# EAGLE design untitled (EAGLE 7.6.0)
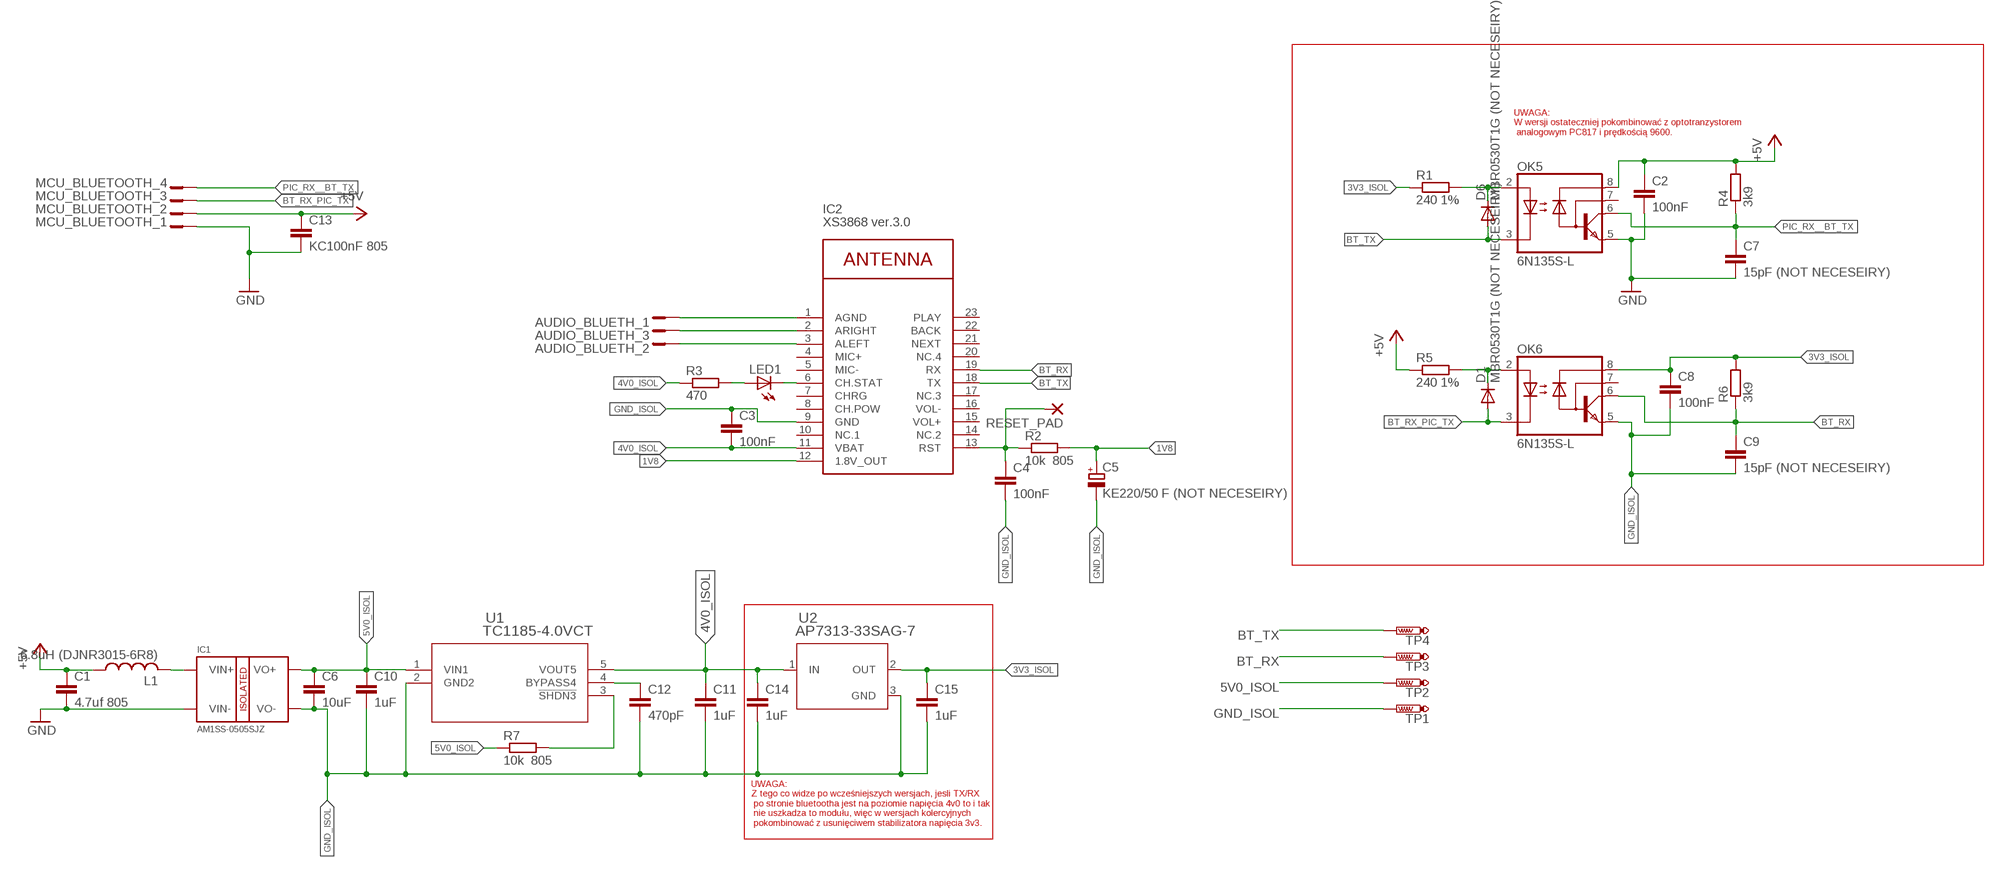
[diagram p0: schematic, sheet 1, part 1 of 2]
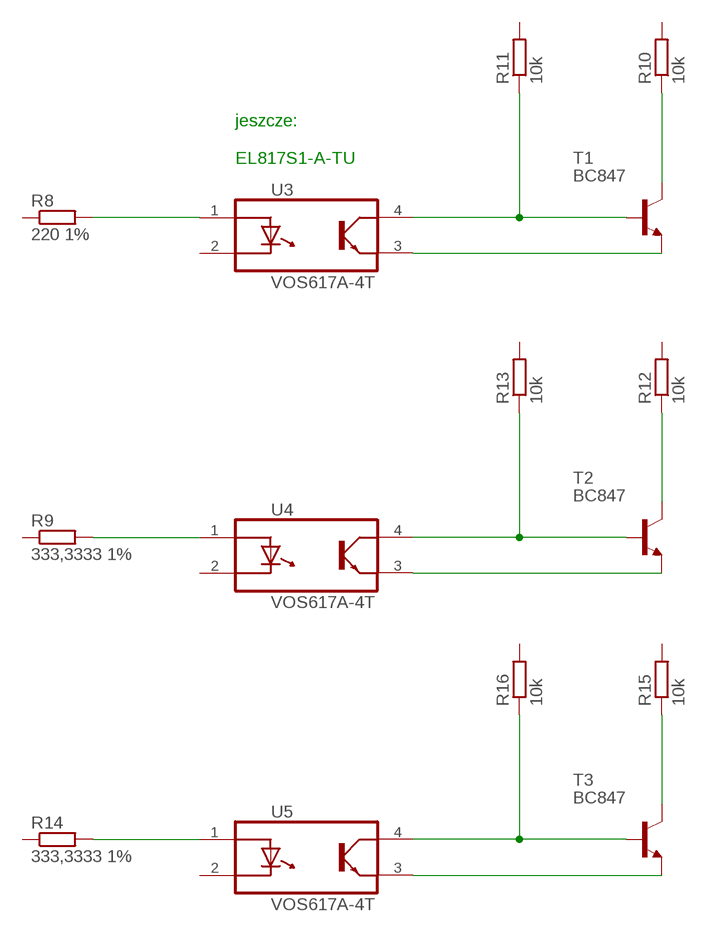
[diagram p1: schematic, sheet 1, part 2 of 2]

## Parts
AUDIO_BLUETH  JST_3_PIN_B3B-PH-KS  [B3B-PH-KS]
C1  4.7uf 805  C-EUC0805  [C0805]
C2  100nF  C-EUC0805  [C0805]
C3  100nF  C-EUC0805  [C0805]
C4  100nF  C-EUC0805  [C0805]
C5  KE220/50 F (NOT NECESEIRY)  CPOL-EUG  [PANASONIC_G]
C6  10uF  C-EUC0805  [C0805]
C7  15pF (NOT NECESEIRY)  C-EUC0805  [C0805]
C8  100nF  C-EUC0805  [C0805]
C9  15pF (NOT NECESEIRY)  C-EUC0805  [C0805]
C10  1uF  C-EUC0805  [C0805]
C11  1uF  C-EUC0805  [C0805]
C12  470pF  C-EUC0805  [C0805]
C13  KC100nF 805  C-EUC0805  [C0805]
C14  1uF  C-EUC0805  [C0805]
C15  1uF  C-EUC0805  [C0805]
D1  MBR0530T1G (NOT NECESEIRY)  MBR0520LT  [SOD123]
D6  MBR0530T1G (NOT NECESEIRY)  MBR0520LT  [SOD123]
IC1  AM1SS-0505SJZ  AM1SS-0503S-NZ  [SIP4]
IC2  XS3868 ver.3.0  WIRELESS-BLUETOOTH-XS3868  [WIRELESS-BLUETOOTH-XS3868]
L1  6.8uH (DJNR3015-6R8)  L-USL3230M  [L3230M]
LED1  LEDSMART-LED  [SMART-LED]
MCU_BLUETOOTH  JST_4_PIN_B4B-PH-KS  [B4B-PH-KS]
OK5  6N135S-L  6N135DIL8-SMD  [DIL8-SMD]
OK6  6N135S-L  6N135DIL8-SMD  [DIL8-SMD]
R1  240 1%  R-EU_M0805  [M0805]
R2  10k 805  R-EU_M0805  [M0805]
R3  470  R-EU_M0805  [M0805]
R4  3k9  R-EU_M0805  [M0805]
R5  240 1%  R-EU_M0805  [M0805]
R6  3k9  R-EU_M0805  [M0805]
R7  10k 805  R-EU_M0805  [M0805]
R8  220 1%  R-EU_M0805  [M0805]
R9  333,3333 1%  R-EU_M0805  [M0805]
R10  10k  R-EU_M0805  [M0805]
R11  10k  R-EU_M0805  [M0805]
R12  10k  R-EU_M0805  [M0805]
R13  10k  R-EU_M0805  [M0805]
R14  333,3333 1%  R-EU_M0805  [M0805]
R15  10k  R-EU_M0805  [M0805]
R16  10k  R-EU_M0805  [M0805]
RESET_PAD  SMD2  [SMD1,27-2,54]
T1  BC847  [SOT23]
T2  BC847  [SOT23]
T3  BC847  [SOT23]
TP1  PTR1B1,27  [B1,27]
TP2  PTR1B1,27  [B1,27]
TP3  PTR1B1,27  [B1,27]
TP4  PTR1B1,27  [B1,27]
U1  TC1185-4.0VCT  TC1185-X.XXCT713SOT-23-5_MC-M  [SOT-23-5_MC-M]
U2  AP7313-33SAG-7  [SOT-23]
U3  VOS617A-4T  [SOIC127P700X210-4N]
U4  VOS617A-4T  [SOIC127P700X210-4N]
U5  VOS617A-4T  [SOIC127P700X210-4N]

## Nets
1V8: C5.+ IC2.12(1.8V_OUT) R2.2
3V3_ISOL: C8.1 C15.1 OK6.8(VCC) R1.1 R6.2 U2.2(OUT)
4V0_ISOL: C3.2 C11.1 C14.1 IC2.11(VBAT) R3.1 U1.5(VOUT5) U2.1(IN)
5V0_ISOL: C6.1 C10.1 IC1.P$4(VO+) R7.1 TP2.TP U1.1(VIN1)
+5V: C1.1 C2.1 C13.1 L1.1 MCU_BLUETOOTH.P$2 OK5.8(VCC) R4.2 R5.1
AGND: AUDIO_BLUETH.P$1 IC2.1(AGND)
BT_LED: IC2.6(CH.STAT) LED1.B(C)
BT_RX: C9.1 IC2.19(RX) OK6.6(VO) R6.1 TP3.TP
BT_RX_PIC_TX: D1.A MCU_BLUETOOTH.P$3 OK6.3(C)
BT_TX: D6.A IC2.18(TX) OK5.3(C) TP4.TP
BTOUT_LEFT: AUDIO_BLUETH.P$2 IC2.3(ALEFT)
BTOUT_RIGHT: AUDIO_BLUETH.P$3 IC2.2(ARIGHT)
GND: C1.2 C2.2 C7.2 C13.2 IC1.P$1(VIN-) MCU_BLUETOOTH.P$1 OK5.5(GND)
GND_ISOL: C3.1 C4.2 C5.- C6.2 C8.2 C9.2 C10.2 C11.2 C12.2 C14.2 C15.2 IC1.P$3(VO-) IC2.9(GND) OK6.5(GND) TP1.TP U1.2(GND2) U2.3(GND)
N$1: IC1.P$2(VIN+) L1.2
N$2: D6.C OK5.2(A) R1.2
N$3: D1.C OK6.2(A) R5.2
N$4: C12.1 U1.4(BYPASS4)
N$5: LED1.A R3.2
N$6: R7.2 U1.3(!SHDN3)
N$7: R8.2 U3.1(A)
N$8: R9.2 U4.1(A)
N$9: R10.1 T1.3(C)
N$10: R11.1 T1.1(B) U3.4(CO)
N$11: T1.2(E) U3.3(E)
N$12: R12.1 T2.3(C)
N$13: R13.1 T2.1(B) U4.4(CO)
N$14: T2.2(E) U4.3(E)
N$15: R14.2 U5.1(A)
N$16: R15.1 T3.3(C)
N$17: R16.1 T3.1(B) U5.4(CO)
N$18: T3.2(E) U5.3(E)
PIC_RX__BT_TX: C7.1 MCU_BLUETOOTH.P$4 OK5.6(VO) R4.1
RST: C4.1 IC2.13(RST) R2.1 RESET_PAD.1(P)
Unconnected: IC2.4(MIC+) IC2.5(MIC-) IC2.7(CHRG) IC2.8(CH.POW) IC2.10(NC.1) IC2.14(NC.2) IC2.15(VOL+) IC2.16(VOL-) IC2.17(NC.3) IC2.20(NC.4) IC2.21(NEXT) IC2.22(BACK) IC2.23(PLAY) OK5.7(VB) OK6.7(VB) R8.1 R9.1 R10.2 R11.2 R12.2 R13.2 R14.1 R15.2 R16.2 U3.2(C) U4.2(C) U5.2(C)

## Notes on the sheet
- jeszcze:
  
  EL817S1-A-TU
- UWAGA:
  W wersji ostateczniej pokombinować z optotranzystorem
   analogowym PC817 i prędkością 9600.
- UWAGA:
  Z tego co widze po wcześniejszych wersjach, jesli TX/RX
   po stronie bluetootha jest na poziomie napięcia 4v0 to i tak
   nie uszkadza to modułu, więc w wersjach kolercyjnych
   pokombinować z usunięciwem stabilizatora napięcia 3v3.

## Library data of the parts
AUDIO_BLUETH = conn-JST:JST_3_PIN_
C1 C13 = rcl:C-EU: CAPACITOR, European symbol
C2-C4 C6-C12 C14 C15 = resistor:C-EU: CAPACITOR, European symbol
C5 = rcl:CPOL-EU: POLARIZED CAPACITOR, European symbol
D1 D6 = diode:MBR0520LT: SCHOTTKY BARRIER RECTIFIER
IC1 = DC-DC_converter:AM1SS
IC2 = diy-modules:WIRELESS-BLUETOOTH-XS3868: Bluetooth Stereo Audio Module based on OVC3860 chip More details available here: http://artofcircuits.com/product/bluetooth-2-0-edr-stereo-audio-ovc3860-module-model-xs-3868 Click here to find device on ebay.com
L1 = rcl:L-US: INDUCTOR, American symbol
LED1 = led:LED: LED
MCU_BLUETOOTH = conn-JST:JST_4_PIN_
OK5 OK6 = optocoupler:6N135: MOTOROLA OPTO COUPLER
R1-R16 = rcl:R-EU_: RESISTOR, European symbol
RESET_PAD = wirepad:SMD2: SMD PAD
T1-T3 = nxp_60:BC847: 45 V, 100 mA NPN general-purpose transistors NPN general-purpose transistor AAL Eindhoven MK
TP1-TP4 = testpad:PTR1: TEST PIN
U1 = TC1185:TC1185-X.XXCT713; MANUFACTURER_PART_NUMBER: TC1185X.XXCT713; VENDOR: Microchip
U2 = AP7313:AP7313-33SAG-7; MANUFACTURER_PART_NUMBER: AP731333SAG7; VENDOR: Diodes Inc
U3-U5 = VOS617A-4T:VOS617A-4T; DESCRIPTION: Optocoupler DC-IN 1-CH Transistor DC-OUT 4-Pin SSOP T/R; DIGI-KEY_PART_NUMBER: VOS617A-4TCT-ND; DIGI-KEY_PURCHASE_URL: https://www.digikey.pl/product-detail/en/vishay-semiconductor-opto-division/VOS617A-4T/VOS617A-4TCT-ND/6596775?utm_source=snapeda&utm_medium=aggregator&utm_campaign=symbol; MF: Vishay Semiconductor; MP: VOS617A-4T; PACKAGE: SSOP-4 Vishay

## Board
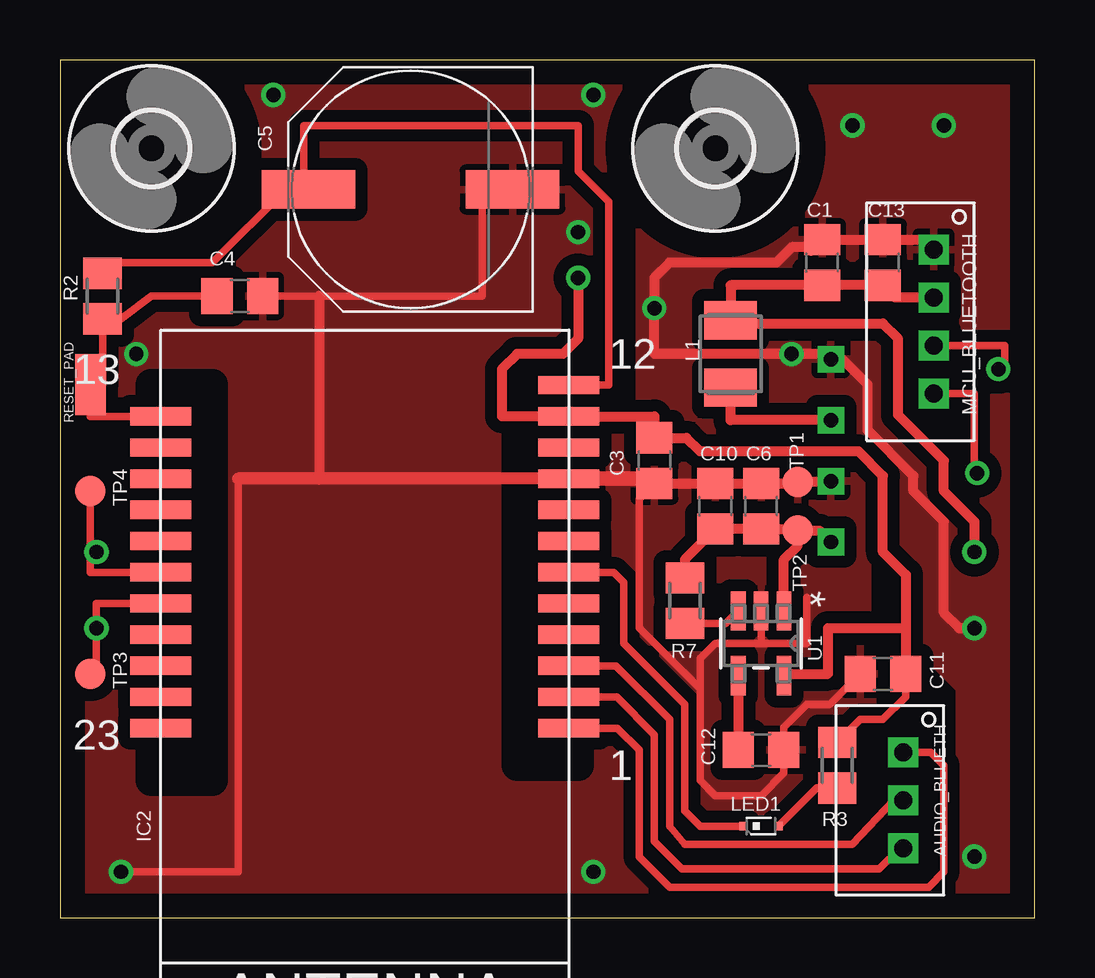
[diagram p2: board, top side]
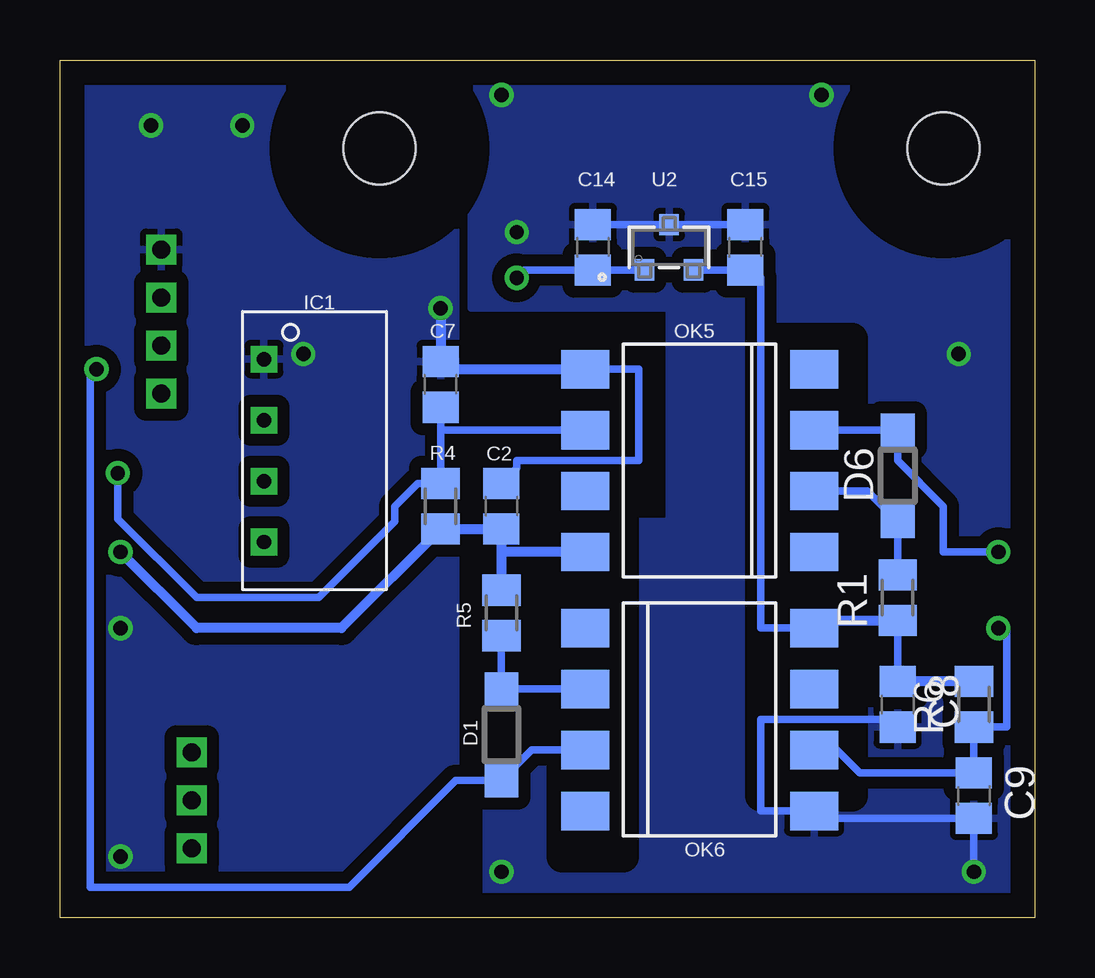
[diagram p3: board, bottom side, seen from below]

Size 40.62 x 35.75 mm. Coordinates in mm from the lower left corner, seen from the top.
Outline: 0,0 40.62,0 40.62,35.75 0,35.75 0,0
Copper layers (1*16): Top 0.035mm / dielectric 1.5mm / Bottom 0.035mm
Design rules "default": minimum track width 10mil, minimum drill 24mil, track to track 8mil, track to pad 8mil, pad to pad 8mil, via to via 8mil, smd to smd 8mil, copper to edge 40mil, drill to drill 8mil, minimum pad ring 10mil, minimum via ring 8mil, stop-mask expansion 4mil, vias tented up to drill 0mil, thermal gap 10mil
tRestrict: area 19.1,6.3 to 21.6,23.5; area 3.8,5.7 to 6.3,22.2
bRestrict: area 17.1,2.5 to 19.7,24.1; area 7.6,5.1 to 11.4,24.1

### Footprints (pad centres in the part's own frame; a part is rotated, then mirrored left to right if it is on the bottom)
B3B-PH-KS = drill 0.75 pad 1.2 square: P$1 -2,1.7; P$2 -4,1.7; P$3 -6,1.7
C0805 = smd 1.3 x 1.5: 1 -0.95,0; 2 0.95,0
PANASONIC_G = smd 3.9 x 1.6: + 4.25,0; - -4.25,0
SOD123 = smd 1.4 x 1.4: A 1.9,0; C -1.9,0
SIP4 = drill 0.6 square: P$1 -0.415,-2.91; P$2 2.125,-2.91; P$3 4.665,-2.91; P$4 7.205,-2.91
WIRELESS-BLUETOOTH-XS3868 = smd 2.54 x 0.762: 1 -8.5,0.995; 2 -8.5,-0.305; 3 -8.5,-1.605; 4 -8.5,-2.905; 5 -8.5,-4.205; 6 -8.5,-5.505; 7 -8.5,-6.805; 8 -8.5,-8.105; 9 -8.5,-9.405; 10 -8.5,-10.705; 11 -8.5,-12.005; 12 -8.5,-13.305; 13 8.5,-12.005; 14 8.5,-10.705; 15 8.5,-9.405; 16 8.5,-8.105; 17 8.5,-6.805; 18 8.5,-5.505; 19 8.5,-4.205; 20 8.5,-2.905; 21 8.5,-1.605; 22 8.5,-0.305; 23 8.5,0.995
L3230M = smd 1.6 x 2.2: 1 -1.4,0; 2 1.4,0
SMART-LED = smd 0.35 x 0.35: A 0,0.725; B 0,-0.725
B4B-PH-KS = drill 0.75 pad 1.2 square: P$1 -2,1.7; P$2 -4,1.7; P$3 -6,1.7; P$4 -8,1.7
DIL8-SMD = smd 1.6 x 2: 1 -3.81,-4.77; 2 -1.27,-4.77; 3 1.27,-4.77; 4 3.81,-4.77; 5 3.81,4.77; 6 1.27,4.77; 7 -1.27,4.77; 8 -3.81,4.77
M0805 = smd 1.3 x 1.6: 1 -0.95,0; 2 0.95,0
SMD1,27-2,54 = smd 1.27 x 2.54: 1 0,0
SOT23 = smd 1 x 1.4: 1 -0.95,-1.1; 2 0.95,-1.1; 3 0,1.1
B1,27 = smd 1.27 x 1.27: TP 0,0
SOT-23-5_MC-M = smd 1.626 x 0.61: 1 -1.346,0.95; 2 -1.346,0; 3 -1.346,-0.95; 4 1.346,-0.95; 5 1.346,0.95
SOT-23 = smd 0.813 x 0.889: 1 -1.025,-0.945; 2 1.025,-0.945; 3 0,0.945
SOIC127P700X210-4N = smd 1.84 x 0.64: 1 -3.085,0.635; 2 -3.085,-0.635; 3 3.085,-0.635; 4 3.085,0.635
3,0 = hole 3: 0,0

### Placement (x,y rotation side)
AUDIO_BLUETH  36.83,8.89 90 top
C1  31.75,27.3 90 top
C2  22.22,17.14 90 bottom
C3  24.77,19.05 90 top
C4  7.49,25.91 0 top
C5  14.61,30.35 180 top
C6  29.21,17.14 90 top
C7  24.77,22.22 90 bottom
C8  5.71,8.89 270 bottom
C9  2.54,5.08 270 bottom
C10  27.3,17.14 90 top
C11  34.29,10.16 180 top
C12  29.21,6.98 0 top
C13  34.29,27.3 90 top
C14  18.41,27.94 90 bottom
C15  12.06,27.94 90 bottom
D1  22.22,7.62 270 bottom
D6  5.71,18.41 90 bottom
IC1  29.21,22.86 270 bottom
IC2  12.7,8.89 180 top
L1  27.94,23.49 270 top
LED1  29.21,3.81 270 top
MCU_BLUETOOTH  38.1,29.84 90 top
OK5  13.97,19.05 90 bottom
OK6  13.97,8.25 270 bottom
R1  5.71,13.34 90 bottom
R2  1.78,25.91 90 top
R3  32.38,6.35 270 top
R4  24.77,17.14 270 bottom
R5  22.22,12.7 270 bottom
R6  2.54,8.89 90 bottom
R7  26.03,13.21 270 top
R8  not placed on the board
R9  not placed on the board
R10  not placed on the board
R11  not placed on the board
R12  not placed on the board
R13  not placed on the board
R14  not placed on the board
R15  not placed on the board
R16  not placed on the board
RESET_PAD  1.27,22.22 180 top
T1  not placed on the board
T2  not placed on the board
T3  not placed on the board
TP1  30.73,18.16 0 top
TP2  30.73,16.13 0 top
TP3  1.27,10.16 0 top
TP4  1.27,17.78 0 top
U1  29.21,11.43 270 top
U2  15.24,27.94 0 bottom
U3  not placed on the board
U4  not placed on the board
U5  not placed on the board
U$2  [3,0]  3.81,32.07 0 top
U$3  [3,0]  27.3,32.07 0 top

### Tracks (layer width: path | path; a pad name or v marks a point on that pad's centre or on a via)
1V8
  Top 0.305: IC2.12 22.86,22.2 22.86,29.84 21.59,31.12 21.59,33.02 10.16,33.02 10.16,30.79 C5.+ 9.4,30.35 6.35,27.3 1.78,27.3 R2.2
3V3_ISOL
  Bottom 0.254: OK6.8 8.88,12.38
  Bottom 0.305: OK6.8 11.43,12.06 11.43,26.67 11.75,26.99 C15.1 U2.2 | C8.1 R1.1
  Bottom 0.406: R6.2 C8.1 | 8.88,12.38 R1.1
4V0_ISOL  (via drill 0.6)
  Top 0.305: R3.1 33.34,8.25 34.29,8.25 35.24,9.2 C11.1
  Top 0.406: v21.59,26.67 21.59,24.13 20.95,23.49 19.05,23.49 18.41,22.86 18.41,20.89 IC2.11 24.77,20.89 C3.2 26.1,20 26.67,19.43 33.27,19.43 34.29,18.41 34.29,15.24 35.24,14.29 35.24,12.06 | 35.24,12.06 C11.1 | U1.5 30.24,10.16 32,10.16 32,12.06 35.24,12.06
  Bottom 0.305: v21.59,26.67 21.27,26.99 C14.1 U2.1
5V0_ISOL
  Top 0.406: TP2.TP 30.67,16.2 C6.1 C10.1 26.03,14.93 R7.1 | TP2.TP 31.65,16.13 IC1.P$4 | U1.1 30.16,14.92 30.73,15.49 TP2.TP
+5V  (via drill 0.6)
  Top 0.406: MCU_BLUETOOTH.P$2 34.8,25.84 C13.1 C1.1 27.94,26.35 L1.1 27.94,24.77 34.29,24.77 34.92,24.13 34.92,20.95 36.83,19.05 36.83,17.78 38.1,16.51 v38.1,15.24
  Bottom 0.406: 22.22,15.24 C2.1 R4.2 28.89,12.06 34.92,12.06 v38.1,15.24 | 22.22,15.24 R5.1 | OK5.8 22.22,15.24
AGND
  Top 0.305: AUDIO_BLUETH.P$1 36.29,6.89 36.83,6.35 36.83,1.9 36.2,1.27 25.4,1.27 24.13,2.54 24.13,6.98 23.22,7.89 IC2.1
BT_LED
  Top 0.305: IC2.6 23.07,14.39 23.49,13.97 23.49,11.43 26.03,8.89 26.03,4.45 26.67,3.81 LED1.B
BT_RX  (via drill 0.6)
  Top 0.305: IC2.19 1.52,13.09 v1.52,12.06 1.52,10.41 TP3.TP
  Bottom 0.305: OK6.6 8.25,6.98 7.3,6.03 C9.1 R6.1 1.17,7.94 1.17,12.06 v1.52,12.06
BT_RX_PIC_TX  (via drill 0.6)
  Top 0.305: MCU_BLUETOOTH.P$3 39.37,23.84 39.37,22.86 v39.1,22.86
  Bottom 0.305: OK6.3 20.96,6.98 D1.A 24.12,5.72 28.58,1.27 39.37,1.27 39.37,22.59 arc90 v39.1,22.86
BT_TX  (via drill 0.6)
  Top 0.305: IC2.18 1.27,14.39 1.27,15.24 | 1.27,15.24 v1.52,15.24 | TP4.TP 1.27,15.24
  Bottom 0.305: OK5.3 D6.A 5.71,19.05 3.81,17.14 3.81,15.24 v1.52,15.24
BTOUT_LEFT
  Top 0.305: IC2.3 23.16,10.5 25.4,8.25 25.4,3.81 26.03,3.05 33.02,3.05 34.73,4.89 AUDIO_BLUETH.P$2
BTOUT_RIGHT
  Top 0.305: IC2.2 23.19,9.2 24.77,7.62 24.77,3.17 25.91,2.03 34.14,2.03 35,2.89 AUDIO_BLUETH.P$3
GND  (via drill 0.6)
  Top 0.406: MCU_BLUETOOTH.P$1 35.99,28.26 C13.2 C1.2 | v38.1,12.06 37.46,12.06 36.83,12.7 36.83,16.51 35.56,17.78 35.56,18.41 33.66,20.32 33.66,22.22 32.38,23.49 31.9,23.49 | C1.2 31.3,27.8 | IC1.P$1 31.9,23.49 | 31.9,23.49 24.77,23.49 v24.77,25.4 24.77,26.67 25.4,27.3 29.84,27.3 30.48,27.94 31.44,27.94 C1.2
  Bottom 0.305: C2.2 21.59,18.73 21.59,19.05 16.51,19.05 16.51,22.86 OK5.5
  Bottom 0.406: OK5.5 25.09,22.86 C7.2 v24.77,25.4
  other vias: 36.83,33.02 33.02,33.02 38.1,2.54 30.48,23.49
  pour Top (isolate 0.508): 24.13,38.1 43.18,38.1 43.18,-1.27 37.46,-1.27 37.46,9.52 34.29,12.7 34.29,19.68 24.13,19.68
  pour Bottom (isolate 0.508): 41.91,-1.27 24.13,-1.27 24.13,36.83 41.91,36.83
GND_ISOL  (via drill 0.6)
  Top 0.305: C4.2 10.79,25.91 17.59,25.91 17.59,30.35 C5.- | 7.43,18.29 7.43,1.9 v2.54,1.9 | C10.2 C3.1 24.13,17.45 24.13,12.06 26.67,9.52 | 26.67,9.52 26.67,5.71 27.3,5.08 29.21,5.08 30.16,6.03 C12.2 30.16,7.93 31.12,8.89 32.07,8.89 C11.2 | 26.67,9.52 26.67,10.79 27.3,11.43 29.21,11.43 | 31.12,13.34 31.12,11.43 29.21,11.43 | U1.2 29.21,11.43
  Top 0.406: 10.79,25.91 10.79,18.29 | C3.1 C6.2 30.67,18.09 TP1.TP 32.09,18.16 IC1.P$3
  Top 0.508: IC2.9 10.79,18.29 7.43,18.29
  Top 0.61: IC2.9 24.77,18.29 C3.1
  Bottom 0.305: C8.2 arc-90 6.03,8.25 11.43,8.25 11.43,4.45 OK6.5 8.88,4.13 C9.2 v2.54,1.9 | C14.2 U2.3 C15.2
  other vias: 21.59,28.58 3.17,23.49 8.89,34.29 22.22,34.29 22.22,1.9
  pour Top (isolate 0.508): -3.81,-3.18 -3.81,38.1 23.49,38.1 23.49,19.05 33.66,19.05 33.66,12.06 36.83,8.89 36.83,-3.18
  pour Bottom (isolate 0.508): -2.54,-1.91 -2.54,36.83 23.49,36.83 23.49,25.4 15.24,25.4 15.24,16.51 25.4,16.51 25.4,15.24 22.86,15.24 22.86,-1.91
N$1
  Top 0.406: IC1.P$2 27.94,20.73 L1.2
N$2
  Bottom 0.305: OK5.2 6.98,17.78 D6.C R1.2
N$3
  Bottom 0.305: OK6.2 D1.C R5.2
N$4
  Top 0.406: U1.4 C12.1
N$5
  Top 0.305: LED1.A 31.52,5.4 R3.2
N$6
  Top 0.305: R7.2 27.74,12.26 U1.3
N$7  (1 unrouted)
N$8  (1 unrouted)
N$9  (1 unrouted)
N$10  (2 unrouted)
N$11  (1 unrouted)
N$12  (1 unrouted)
N$13  (2 unrouted)
N$14  (1 unrouted)
N$15  (1 unrouted)
N$16  (1 unrouted)
N$17  (2 unrouted)
N$18  (1 unrouted)
PIC_RX__BT_TX  (via drill 0.6)
  Top 0.305: MCU_BLUETOOTH.P$4 38.1,21.84 38.1,18.64 v38.21,18.53
  Bottom 0.305: C7.1 24.77,20.32 | 24.77,20.32 R4.1 25.72,18.09 26.67,17.14 26.67,16.51 29.84,13.34 34.92,13.34 38.21,16.62 v38.21,18.53 | OK5.6 24.77,20.32
RST
  Top 0.305: C4.1 3.81,25.91 2.54,24.96 R2.1 1.78,22.22 RESET_PAD.1 1.27,20.89 IC2.13

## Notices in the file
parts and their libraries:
diy-modules: Released under the Creative Commons Attribution 4.0 International License: http://creativecommons.org/licenses/by/4.0
